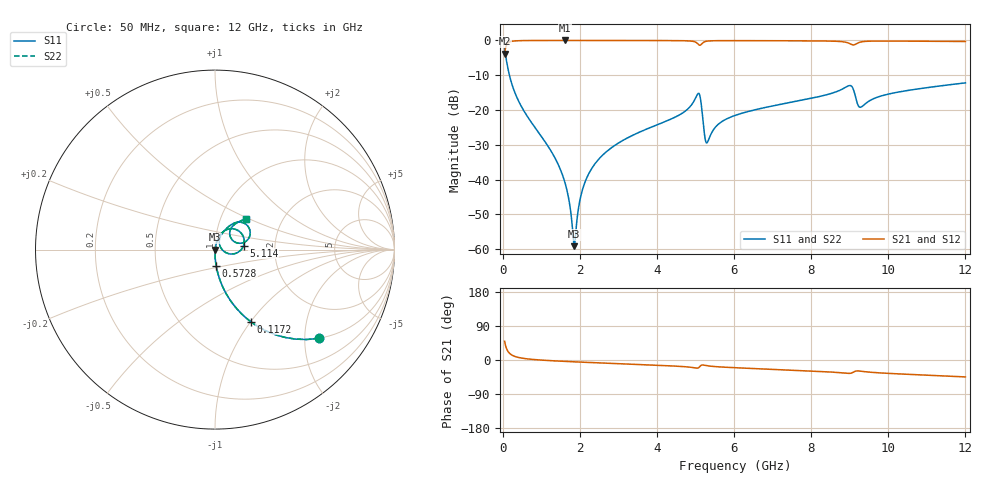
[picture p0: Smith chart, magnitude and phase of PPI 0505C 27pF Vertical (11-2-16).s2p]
# GHz S MA R 50
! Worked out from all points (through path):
!   1601 points, 50 MHz to 12 GHz, reference 50 ohm
!   highest |S21| = -0.01 dB at 1.618 GHz (marker M1); lowest = -3.8 dB at 50 MHz (marker M2)
!   group delay of S21, straight-line fit = 11.5 ps
!   lowest |S11| = -59.2 dB at 1.857 GHz (marker M3), VSWR 1.00, Z = 50.1 - j0.00632 ohm
!   |S11| at or under -10 dB: 174.8 MHz to end of sweep
!   |S22| runs from -59.2 to -2.4 dB; largest |S21 - S12| = 0
!   S11 on the Smith chart (normalised r, x): 50 MHz: 1.00, -2.34; 117.2 MHz: 1.00, -1.00; 572.8 MHz: 1.00, -0.19; 5.114 GHz: 1.38, +0.06; 12 GHz: 1.32, +0.48
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0.05  0.7615 -40.5  0.648 49.5  0.648 49.5  0.7615 -40.5
0.1172187  0.4468 -63.7  0.8943 26.2  0.8943 26.2  0.4468 -63.7
0.2367188  0.2373 -76.8  0.971 13.1  0.971 13.1  0.2373 -76.8
0.5728125  0.09258 -85.8  0.995 3.8  0.995 3.8  0.09258 -85.8
1.30475  0.02301 -89.7  0.9987 -2.1  0.9987 -2.1  0.02301 -89.7
1.618437  0.008902 -87.0  0.9988 -3.7  0.9988 -3.7  0.008902 -87.0
1.857438  0.001102 -3.3  0.9988 -4.8  0.9988 -4.8  0.001102 -3.3
2.044156  0.006352 73.9  0.9987 -5.7  0.9987 -5.7  0.006352 73.9
2.275688  0.01342 78.1  0.9985 -6.7  0.9985 -6.7  0.01342 78.1
2.641656  0.02379 78.6  0.9982 -8.2  0.9982 -8.2  0.02379 78.6
4.038312  0.06226 74.1  0.9958 -14.0  0.9958 -14.0  0.06226 74.1
4.986844  0.1428 54.2  0.9533 -20.8  0.9533 -20.8  0.1428 54.2
5.113812  0.1608 8.1  0.8519 -17.2  0.8519 -17.2  0.1608 8.1
5.240781  0.04167 -3.0  0.9587 -14.0  0.9587 -14.0  0.04167 -3.0
5.300531  0.0338 31.4  0.9761 -15.1  0.9761 -15.1  0.0338 31.4
5.584344  0.06181 66.4  0.9916 -18.0  0.9916 -18.0  0.06181 66.4
6.025  0.08343 67.4  0.9928 -20.3  0.9928 -20.3  0.08343 67.4
8.019156  0.148 59.4  0.9847 -29.1  0.9847 -29.1  0.148 59.4
9.005031  0.2249 34.3  0.8983 -35.2  0.8983 -35.2  0.2249 34.3
9.288844  0.1098 36.6  0.9498 -29.5  0.9498 -29.5  0.1098 36.6
10.01331  0.1697 52.7  0.9791 -35.3  0.9791 -35.3  0.1697 52.7
12  0.2453 44.5  0.965 -44.7  0.965 -44.7  0.2453 44.5
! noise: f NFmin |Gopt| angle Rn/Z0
0.05  0.0003669  0.8579  0.9294  0.0005522
1.372  0.003683  0.6519  3.677  0.00201
2.701  0.006138  0.6016  6.829  0.002832
4.031  0.009187  0.6032  9.987  0.004243
5.36  0.02861  0.8092  13.81  0.03078
6.682  0.01394  0.5761  16.28  0.005854
8.012  0.01782  0.5984  19.42  0.00795
9.341  0.05532  0.8279  23.78  0.06481
10.67  0.02163  0.571  25.32  0.008714
12  0.02199  0.5386  27.55  0.008008
